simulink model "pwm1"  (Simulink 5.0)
settings: Solver=ode45  StartTime=0.0  StopTime=.02  MaxStep=1e-6  RelTol=1e-5
libraries: simulink x1

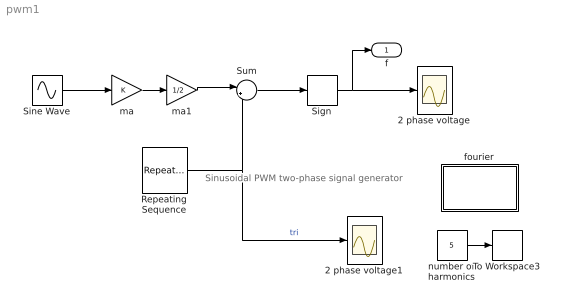
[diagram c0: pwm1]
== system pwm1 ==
  note: Sinusoidal PWM two-phase signal generator
  2 phase voltage : Scope
  2 phase voltage1 : Scope
  Repeating Sequence : simulink/Sources/Repeating Sequence  rep_seq_t="[0  0.5/1000 1/1000]"  rep_seq_y=[1 -1 1]
  Sign : Signum
  Sine Wave : Sin  Frequency=2*pi*50  SampleTime=0
  Sum : Sum  Inputs=|+-
  To Workspace3 : ToWorkspace  VariableName=h  SampleTime=-1  SaveFormat=Array
  fourier : Subsystem
  ma : Gain
  ma1 : Gain  Gain=1/2
  number of harmonics : Constant  Value=5
  f : Outport
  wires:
  ma/1 -> ma1/1
  Sum/1 -> Sign/1
  Repeating Sequence/1 -> Sum/2, 2 phase voltage1/1  "tri"
  Sine Wave/1 -> ma/1
  Sign/1 -> 2 phase voltage/1, f/1
  number of harmonics/1 -> To Workspace3/1
  ma1/1 -> Sum/1

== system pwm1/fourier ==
  note: To obtain the Fourier decomposition of a periodic signal: a) run a simulation for one period duration b) Specify the fundamental frequency c) Specify the number of harmonics
